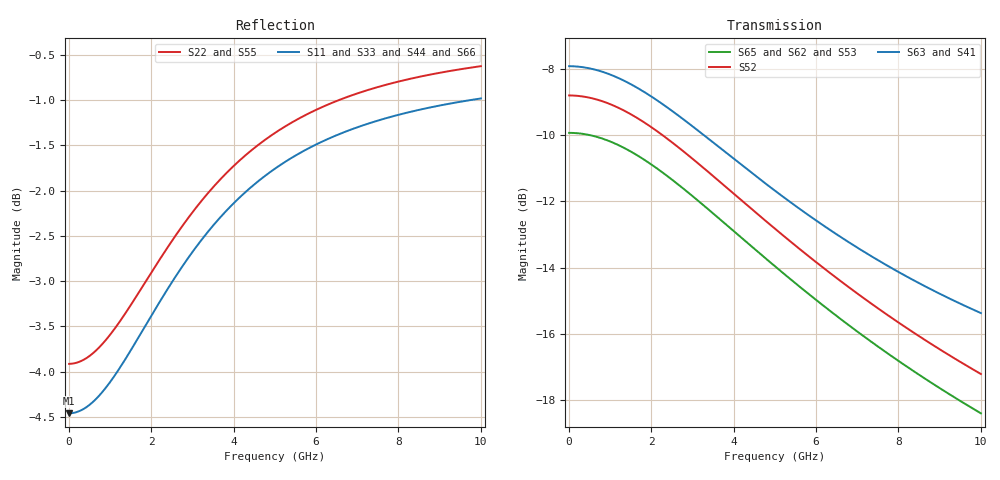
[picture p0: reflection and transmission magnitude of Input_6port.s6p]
! Created Tue Nov 10 08:50:17 2020
# ghz S ma R 50
! 6 Port Network Data from SP1.SP block
! freq  magS11  angS11  magS12  angS12  magS13  angS13  magS14  angS14
!  magS15  angS15  magS16  angS16
!  magS21  angS21  magS22  angS22
!  magS23  angS23  magS24  angS24  magS25  angS25  magS26  angS26
!  magS31  angS31  magS32  angS32  magS33  angS33  magS34  angS34
!  magS35  angS35  magS36  angS36
!  magS41  angS41  magS42  angS42
!  magS43  angS43  magS44  angS44  magS45  angS45  magS46  angS46
!  magS51  angS51  magS52  angS52  magS53  angS53  magS54  angS54
!  magS55  angS55  magS56  angS56
!  magS61  angS61  magS62  angS62
!  magS63  angS63  magS64  angS64  magS65  angS65  magS66  angS66
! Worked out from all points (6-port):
!   1000 points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, 10 MHz to 10 GHz, reference 50 ohm
!   strongest paths, dB at 10 MHz, 2.51 GHz, 5.01 GHz, 7.51 GHz, 10 GHz:
!     S63: -7.9, -9.3, -11.7, -13.8, -15.4
!     S41: -7.9, -9.3, -11.7, -13.8, -15.4
!     S52: -8.8, -10.2, -12.8, -15.2, -17.2
!     S65: -9.9, -11.4, -14.0, -16.4, -18.4
!     S62: -9.9, -11.4, -14.0, -16.4, -18.4
!     S53: -9.9, -11.4, -14.0, -16.4, -18.4
!   lowest |S11| = -4.5 dB at 10 MHz (marker M1), VSWR 3.98, Z = 12.6 + j0.00209 ohm
!   |S11| at or under -10 dB: nowhere
